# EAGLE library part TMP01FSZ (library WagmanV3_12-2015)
Low Power Programmable Temperature Controller
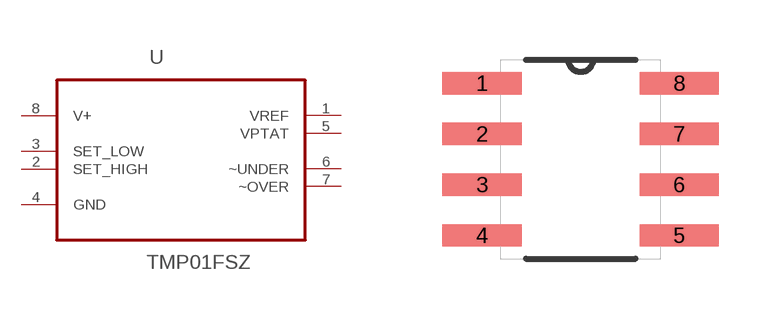
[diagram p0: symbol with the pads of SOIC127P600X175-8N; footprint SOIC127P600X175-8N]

Designator prefix U

## TMP01FSZ (MPN: TMP01FSZ; OC_FARNELL: 1079393; OC_NEWARK: 96K2115; PACKAGE: SOIC-8; SUPPLIER: Analog Devices)  [SOIC127P600X175-8N]
1  VREF  out
2  SET_HIGH  in
3  SET_LOW  in
4  GND  pas
5  VPTAT  out
6  ~UNDER  out
7  ~OVER  out
8  V+  pwr

## Footprint SOIC127P600X175-8N (pad centres in mm)
smd 1.981 x 0.559: 1 -2.464,1.905; 2 -2.464,0.635; 3 -2.464,-0.635; 4 -2.464,-1.905; 5 2.464,-1.905; 6 2.464,-0.635; 7 2.464,0.635; 8 2.464,1.905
